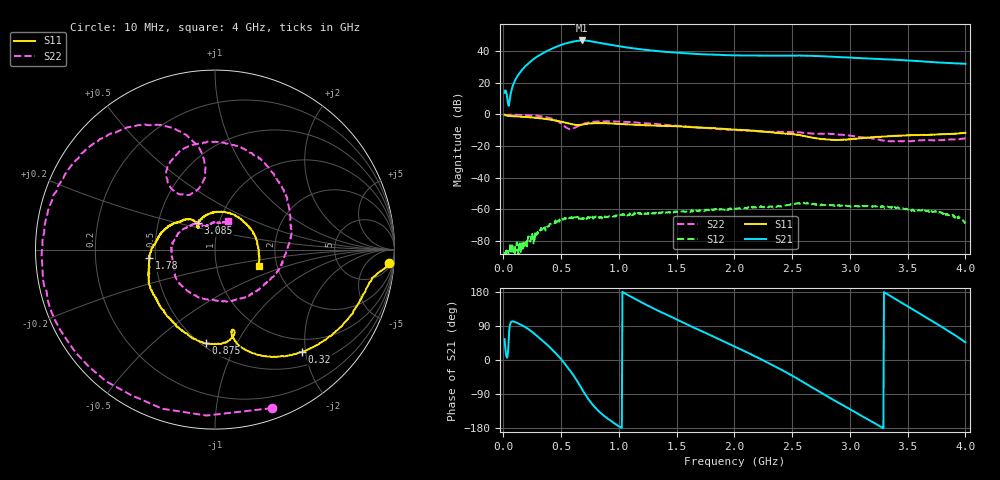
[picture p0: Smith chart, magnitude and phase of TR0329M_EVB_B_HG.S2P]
!Agilent Technologies,E5071C,MY46523237,B.13.01
!Date: Thu Jul 14 13:06:53 2022
!Data & Calibration Information:
!Freq	S11:SOLT2(ON)	S21:SOLT2(ON)	S12:SOLT2(ON)	S22:SOLT2(ON)
!PortZ  Port1:50+j0  Port2:50+j0
!Above PortZ is port z conversion or system Z0 setting when saving the data.
!When reading, reference impedance value at option line is always used.
# Hz S dB R 50
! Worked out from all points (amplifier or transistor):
!   799 points, 10 MHz to 4 GHz, reference 50 ohm
!   highest |S21| = 46.7 dB at 680 MHz (marker M1)
!   |S21| within 3 dB of that: 492.8 MHz to 950.3 MHz (457.5 MHz wide, 63.4 % of centre)
!   unconditionally stable (mu >= 1): start of sweep to end of sweep
!   at 675 MHz: K = 2.88, MAG = 48.9 dB, |S12| = -66.2 dB
!   at 2.005 GHz: K = 5.38, MAG = 38.2 dB, |S12| = -59.7 dB
!   at 4 GHz: K = 28.47, MAG = 32.3 dB, |S12| = -67.9 dB
!   S11 on the Smith chart (normalised r, x): 10 MHz: 9, -22; 320 MHz: 0.74, -1.93; 875 MHz: 0.53, -0.76; 1.78 GHz: 0.46, -0.05; 3.085 GHz: 0.80, +0.24; 4 GHz: 1.61, -0.31
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1e7  -0.27 -4.4  13.62 55.3  -87.05 -173.0  -0.55 -70.3
1.9e8  -1.65 -30.7  30.41 86.6  -82.76 133.2  -0.54 159.0
3.2e8  -2.52 -49.7  37.72 55.9  -73.43 129.6  -1.21 132.2
4.45e8  -3.88 -66.8  42.26 20.3  -68.89 104.0  -3.52 105.0
5.5e8  -5.58 -77.2  45.00 -17.1  -65.53 75.0  -8.70 101.9
6.15e8  -6.62 -78.5  46.08 -44.6  -65.08 59.1  -8.69 123.0
6.75e8  -6.64 -76.6  46.64 -74.4  -66.17 47.6  -6.56 124.2
6.8e8  -6.56 -76.6  46.66 -76.8  -65.95 54.6  -6.43 124.1
7.2e8  -6.08 -78.7  46.49 -96.5  -66.19 51.6  -5.48 119.9
7.7e8  -5.67 -83.6  45.98 -117.1  -64.66 53.3  -4.86 111.6
8.75e8  -5.60 -95.7  44.58 -148.3  -65.26 46.9  -4.47 95.2
1.075e9  -6.40 -115.1  42.16 171.8  -63.77 34.7  -4.92 67.3
1.34e9  -7.23 -136.7  39.86 129.8  -62.64 20.7  -6.29 34.0
1.54e9  -7.68 -153.6  38.79 101.2  -61.51 9.9  -7.43 8.9
1.78e9  -8.62 -172.8  37.80 67.2  -60.66 0.4  -8.82 -22.1
2.005e9  -9.76 170.5  37.25 35.1  -59.72 -9.0  -9.96 -52.8
2.365e9  -11.68 144.5  37.07 -19.3  -58.28 -26.1  -10.98 -107.4
2.67e9  -14.58 125.4  36.91 -72.0  -56.99 -54.6  -12.15 -158.5
3.085e9  -15.18 122.8  35.53 -144.6  -58.38 -72.7  -14.32 135.1
3.335e9  -13.87 98.7  34.68 171.8  -58.62 -82.5  -17.01 112.1
3.655e9  -13.03 47.4  33.27 112.9  -61.06 -95.1  -16.36 91.3
4e9  -11.71 -20.3  31.89 46.7  -67.87 -79.7  -15.18 66.0
